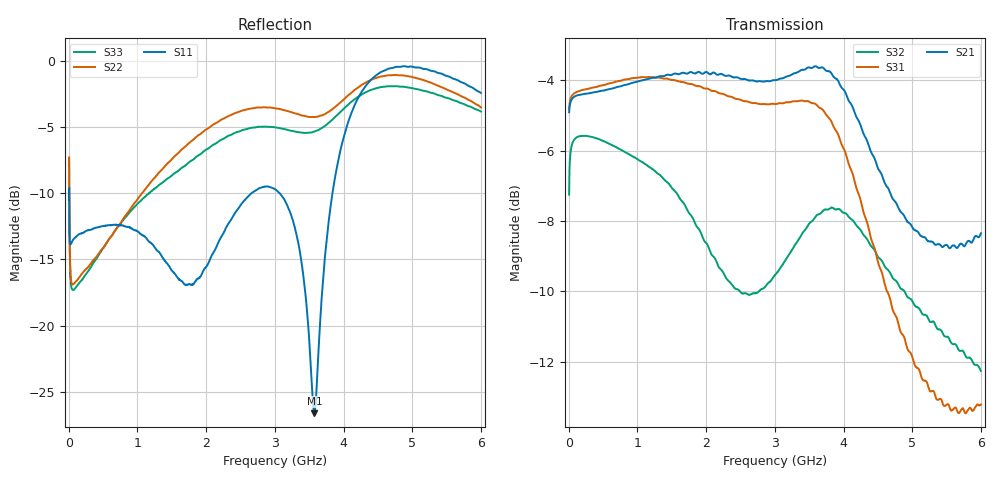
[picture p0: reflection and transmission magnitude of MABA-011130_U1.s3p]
!Agilent Technologies,E5071C,MY46110647,A.11.31
!Date: Fri Mar 25 09:47:41 2022 DD
!Data & Calibration Information:
!MABA-011130 soldered onto PT-0028476 with SMA connectors, Calibration PCB, Port1 (pin1) Port2 (pin2) Port3 (pin3)
!Freq	S11:SOLT3(ON)	S12:SOLT3(ON)	S13:SOLT3(ON)
!	S21:SOLT3(ON)	S22:SOLT3(ON)	S23:SOLT3(ON)
!	S31:SOLT3(ON)	S32:SOLT3(ON)	S33:SOLT3(ON)
!PortZ  Port1:50+j0  Port2:50+j0  Port3:50+j0
!Above PortZ is port z conversion or system Z0 setting when saving the data.
!When reading, reference impedance value at option line is always used.
# Hz S MA R 50
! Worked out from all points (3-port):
!   1200 points, 5 MHz to 6 GHz, reference 50 ohm
!   strongest paths, dB at 5 MHz, 1.505 GHz, 3.005 GHz, 4.505 GHz, 6 GHz:
!     S21: -4.9, -3.8, -4.0, -6.5, -8.3
!     S31: -4.8, -4.0, -4.7, -9.2, -13.2
!     S32: -7.2, -7.1, -9.5, -9.0, -12.3
!   lowest |S11| = -26.6 dB at 3.575 GHz (marker M1), VSWR 1.10, Z = 48.5 - j4.38 ohm
!   |S11| at or under -10 dB: 5.582 MHz to 2.661 GHz (2.655 GHz wide, 199 % of centre); 3.071 GHz to 3.839 GHz (768.2 MHz wide, 22.2 % of centre)
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5000000  0.3304 71.4  0.5645 -164.4  0.5709 15.3
         0.5685 -164.3  0.4315 104.0  0.4343 36.6
         0.5749 15.3  0.4343 36.6  0.4271 103.6
7.5e7  0.2129 2.7  0.598 175.9  0.6045 -3.6
       0.598 175.9  0.1443 23.0  0.519 0.3
       0.6045 -3.7  0.5192 0.3  0.1368 18.4
1.245e9  0.1988 -114.7  0.6409 78.5  0.6369 -96.5
         0.6369 78.8  0.3601 -56.7  0.4734 -66.5
         0.637 -97.5  0.4699 -66.1  0.3277 -90.8
2.115e9  0.1903 -97.3  0.6421 4.7  0.6076 -169.3
         0.6475 5.2  0.5762 -101.4  0.3554 -109.0
         0.6098 -169.3  0.3538 -108.6  0.4831 -119.9
3.005e9  0.3273 -138.7  0.6333 -68.0  0.5803 115.7
         0.6316 -68.7  0.6607 -143.9  0.3419 -135.4
         0.5841 115.4  0.3341 -136.4  0.5595 -151.4
3.575e9  0.04679 -105.8  0.6646 -120.1  0.5755 59.0
         0.6607 -120.5  0.6122 -146.1  0.4095 -169.3
         0.5854 59.1  0.4017 -170.2  0.5397 -153.0
3.825e9  0.2979 -49.1  0.649 -145.2  0.5419 31.8
         0.6457 -146.4  0.6509 -140.3  0.4231 170.9
         0.5511 31.0  0.4164 170.0  0.5942 -149.7
4.21e9  0.7209 -80.2  0.5604 177.8  0.4365 -8.4
        0.5553 177.1  0.7905 -138.7  0.3943 140.8
        0.4377 -9.1  0.3902 140.4  0.7299 -152.8
4.785e9  0.9471 -116.8  0.4204 138.0  0.2885 -51.7
         0.4188 138.0  0.8813 -149.8  0.3213 106.8
         0.2881 -51.3  0.3255 106.9  0.7994 -168.0
6e9  0.755 -174.0  0.3717 71.7  0.2138 -109.5
     0.3825 72.0  0.6659 159.6  0.241 49.6
     0.2183 -108.6  0.2438 49.1  0.6423 140.9
